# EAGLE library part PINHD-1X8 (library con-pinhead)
PIN HEADER
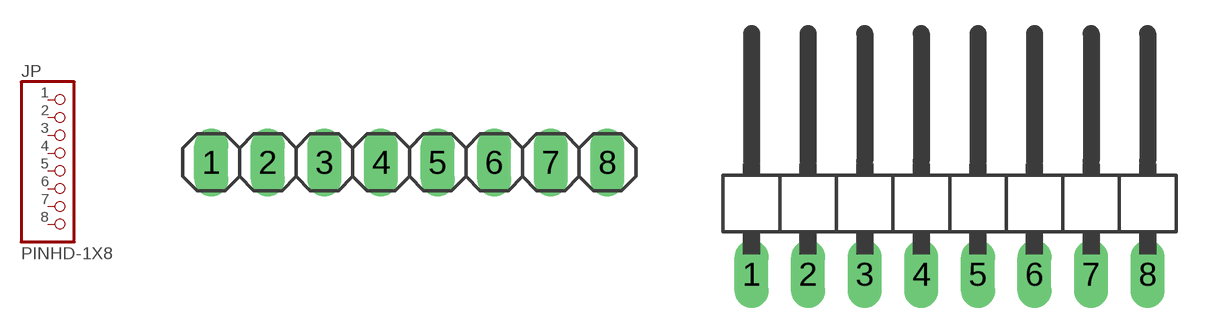
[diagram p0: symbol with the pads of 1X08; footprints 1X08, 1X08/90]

Designator prefix JP

## PINHD-1X8_2.54  [1X08]
1  1  pas
2  2  pas
3  3  pas
4  4  pas
5  5  pas
6  6  pas
7  7  pas
8  8  pas

## PINHD-1X8_2.54-90°  [1X08/90]
Pads as for 1X08

## PINHD-1X8_2.00  [1X08M]
Pads as for 1X08

## PINHD-1X8_2.54-SMD  [1X08SMD]
Pads as for 1X08

## PINHD-1X8_2.54-SMD-90°  [1X08SMD/90]
Pads as for 1X08

## Footprint 1X08 (pad centres in mm)
PIN HEADER - 2.54
drill 1.016 long: 1 -8.89,0; 2 -6.35,0; 3 -3.81,0; 4 -1.27,0; 5 1.27,0; 6 3.81,0; 7 6.35,0; 8 8.89,0

## Footprint 1X08/90 (pad centres in mm)
PIN HEADER - 2.54 90°
drill 1.016 long: 1 -8.89,-3.81; 2 -6.35,-3.81; 3 -3.81,-3.81; 4 -1.27,-3.81; 5 1.27,-3.81; 6 3.81,-3.81; 7 6.35,-3.81; 8 8.89,-3.81

## Footprint 1X08M (pad centres in mm)
PIN HEADER - 2
drill 0.914 square: 1 -7,0
drill 0.914: 2 -5,0; 3 -3,0; 4 -1,0; 5 1,0; 6 3,0; 7 5,0; 8 7,0

## Footprint 1X08SMD (pad centres in mm)
PIN HEADER - 2.54 SMD
smd 1.016 x 3.302: 1 -1.27,1.27; 2 1.27,-1.27; 3 3.81,1.27; 4 6.35,-1.27; 5 8.89,1.27; 6 11.43,-1.27; 7 13.97,1.27; 8 16.51,-1.27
